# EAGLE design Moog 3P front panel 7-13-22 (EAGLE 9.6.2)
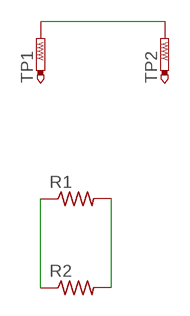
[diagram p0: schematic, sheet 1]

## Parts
R1  R-US_M3216  [M3216]
R2  R-US_M3216  [M3216]
TP1  PTR1B1,27  [B1,27]
TP2  PTR1B1,27  [B1,27]

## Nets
N$1: TP1.TP TP2.TP
N$2: R1.1 R2.1
N$3: R1.2 R2.2

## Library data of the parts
R1 R2 = rcl:R-US_: RESISTOR, American symbol; SPICEPREFIX: R
TP1 TP2 = testpad-CL:PTR1: TEST PIN

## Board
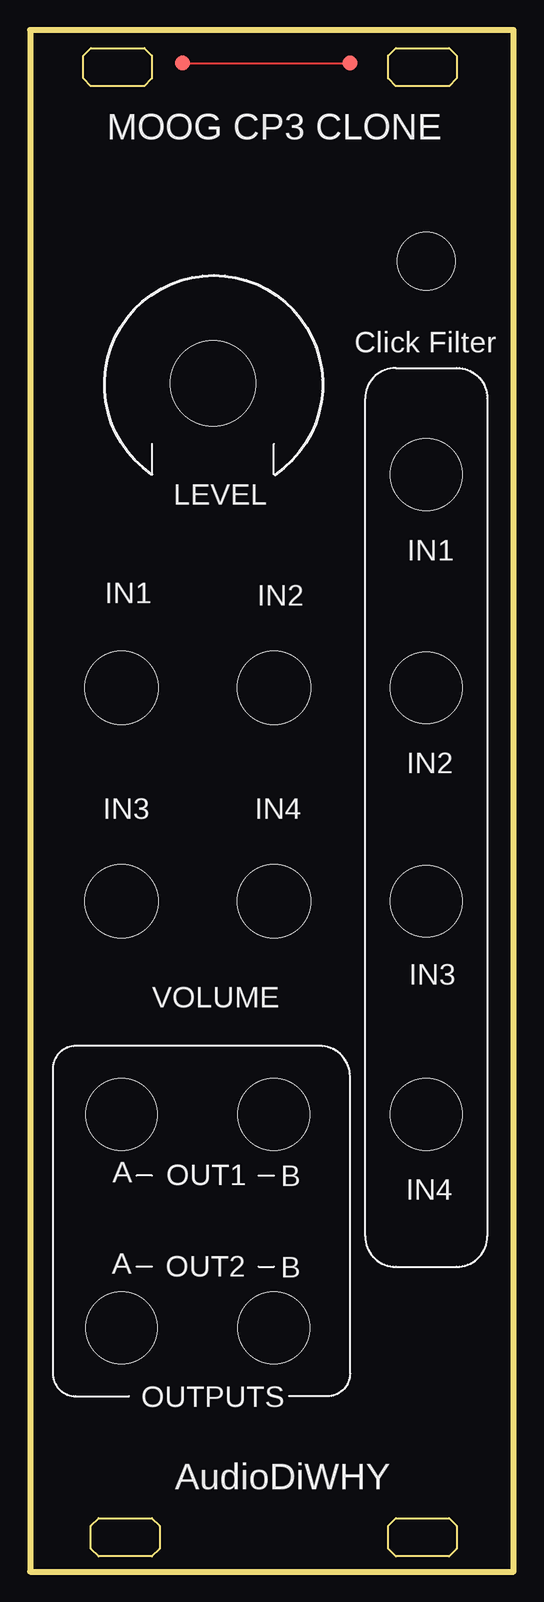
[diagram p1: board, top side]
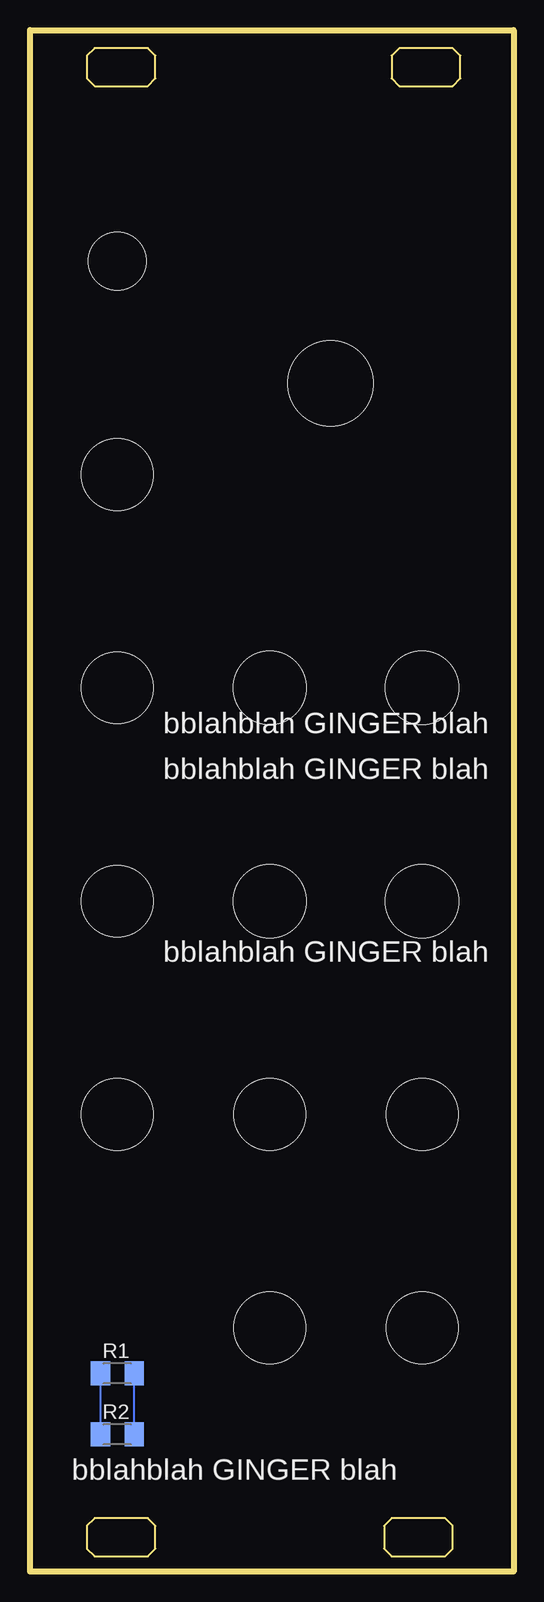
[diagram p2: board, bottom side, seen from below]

Size 40.3 x 128.5 mm. Coordinates in mm from the lower left corner, seen from the top.
Outline: 0,0 40.3,0 40.3,128.5 0,128.5 0,0
Copper layers (1*16): Top 0.035mm / dielectric 1.5mm / Bottom 0.035mm
Design rules "default": minimum track width 6mil, minimum drill 0.35mm, track to track 6mil, track to pad 6mil, pad to pad 6mil, via to via 6mil, smd to smd 6mil, copper to edge 40mil, drill to drill 6mil, minimum pad ring 10mil, minimum via ring 8mil, stop-mask expansion 4mil, vias tented up to drill 0mil, thermal gap 10mil
Holes 5.97 mm at 7.62,20.32 20.32,20.32 7.62,38.1 20.32,38.1 33.02,38.1 33.02,55.88 33.02,73.66 33.02,91.44
Holes 6.1 mm at 7.62,55.88 20.32,55.88 7.62,73.66 20.32,73.66
Holes 4.83 mm at 33.02,109.22
Holes 7.11 mm at 15.24,99.06
Milling: 32 lines

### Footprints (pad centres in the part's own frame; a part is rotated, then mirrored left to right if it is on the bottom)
M3216 = smd 1.6 x 2: 1 -1.4,0; 2 1.4,0
B1,27 = smd 1.27 x 1.27: TP 0,0

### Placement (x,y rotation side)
R1  33.02,16.51 0 bottom
R2  33.02,11.43 0 bottom
TP1  12.7,125.73 0 top
TP2  26.67,125.73 0 top

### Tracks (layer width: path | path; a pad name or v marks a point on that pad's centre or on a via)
N$1
  Top 0.152: TP1.TP TP2.TP
N$2
  Bottom 0.152: R2.1 R1.1
N$3
  Bottom 0.152: R2.2 R1.2

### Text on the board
tNames: MOOG CP3 CLONE | Click Filter | LEVEL | IN1 | IN1 | IN2 | IN2 | IN3 | IN4 | IN3 | VOLUME | A | OUT1 | B | IN4 | A | OUT2 | B | OUTPUTS | AudioDiWHY
bNames: bblahblah GINGER blah | bblahblah GINGER blah | bblahblah GINGER blah | bblahblah GINGER blah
